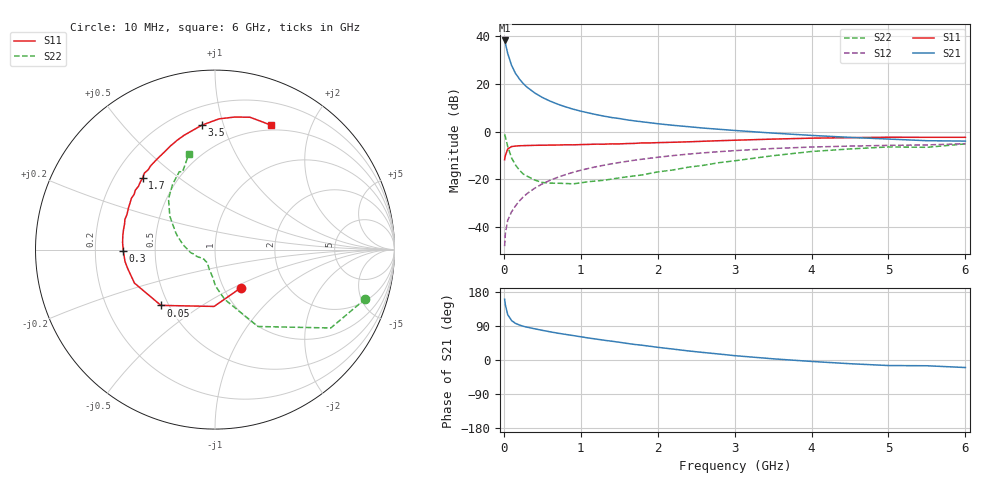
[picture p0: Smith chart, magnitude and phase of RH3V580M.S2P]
! SIEMENS Small Signal Semiconductors
! BFR106
! Si NPN RF Bipolar Junction Transistor in SOT23
! VCE = 3.5 V  IC = 80 mA
! Common Emitter S-Parameters:  August  1996
# GHz  S  MA  R  50
!  f  S11  S21  S12  S22
! GHz  MAG  ANG  MAG  ANG  MAG  ANG  MAG  ANG
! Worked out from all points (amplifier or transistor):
!   36 points, 10 MHz to 6 GHz, reference 50 ohm
!   highest |S21| = 38.2 dB at 10 MHz (marker M1)
!   |S21| within 3 dB of that: start of sweep to 32.74 MHz
!   unconditionally stable (mu >= 1): 190.1 MHz to 2.488 GHz; 5.432 GHz to end of sweep
!   at 250 MHz: K = 1.04, MAG = 22.5 dB, |S12| = -27.4 dB
!   at 1.4 GHz: K = 1.06, MAG = 8.2 dB, |S12| = -13.5 dB
!   at 6 GHz: K = 1.00, MAG = 0.4 dB, |S12| = -5.1 dB
!   S11 on the Smith chart (normalised r, x): 10 MHz: 1.20, -0.55; 50 MHz: 0.45, -0.35; 300 MHz: 0.32, -0.01; 1.7 GHz: 0.32, +0.37; 3.5 GHz: 0.31, +0.85; 6 GHz: 0.44, +1.45
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0.01  0.2572 -56.3  80.88 160.5  0.004 78.3  0.882 -18.1
0.02  0.3167 -90.9  70.24 145.4  0.0074 70.9  0.7791 -34.1
0.05  0.4329 -134.1  43.42 119.9  0.0138 61.4  0.4908 -60.8
0.1  0.4859 -157.4  24.49 104.2  0.0209 64.9  0.2826 -79.0
0.15  0.4974 -167.5  16.75 96.8  0.0277 68.2  0.2019 -89.4
0.2  0.5057 -172.3  12.77 92.6  0.035 71.1  0.1578 -94.1
0.25  0.5082 -176.8  10.21 89.1  0.0426 71.8  0.1302 -100.7
0.3  0.511 -179.3  8.545 86.7  0.0501 73.2  0.1175 -105.3
0.4  0.5163 175.7  6.469 82.4  0.0652 73.7  0.0969 -113.3
0.5  0.5193 171.5  5.193 78.3  0.0805 73.3  0.0862 -119.8
0.6  0.5216 167.8  4.353 74.5  0.0957 72.4  0.0836 -124.2
0.7  0.5238 164.1  3.756 70.8  0.1104 71.5  0.0831 -129.8
0.8  0.5295 161.4  3.305 67.7  0.1255 70.0  0.0821 -135.1
1.1  0.5399 151.3  2.46 58.1  0.1696 65.9  0.0897 -145.7
1.4  0.5538 143.2  1.973 49.6  0.2117 61.3  0.1014 -155.7
1.7  0.5666 135.4  1.674 41.1  0.252 56.6  0.1183 -166.9
2.2  0.5984 122.8  1.354 28.8  0.3148 48.6  0.1574 177.9
2.8  0.6449 109.0  1.118 15.7  0.3803 38.9  0.224 159.9
3.5  0.6969 96.1  0.93 3.1  0.4432 28.2  0.3132 143.5
4.5  0.7468 81.5  0.757 -9.8  0.4971 13.7  0.4337 123.0
5.5  0.759 69.6  0.645 -15.2  0.5266 4.5  0.469 112.7
6  0.7597 65.7  0.633 -19.9  0.5591 -2.5  0.5537 105.2
